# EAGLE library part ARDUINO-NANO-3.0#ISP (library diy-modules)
Arduino Nano 3.0 (and compatible devices) with ISP pads More details available here: https://www.arduino.cc/en/Main/ArduinoBoardNano Click here to find device on ebay.com
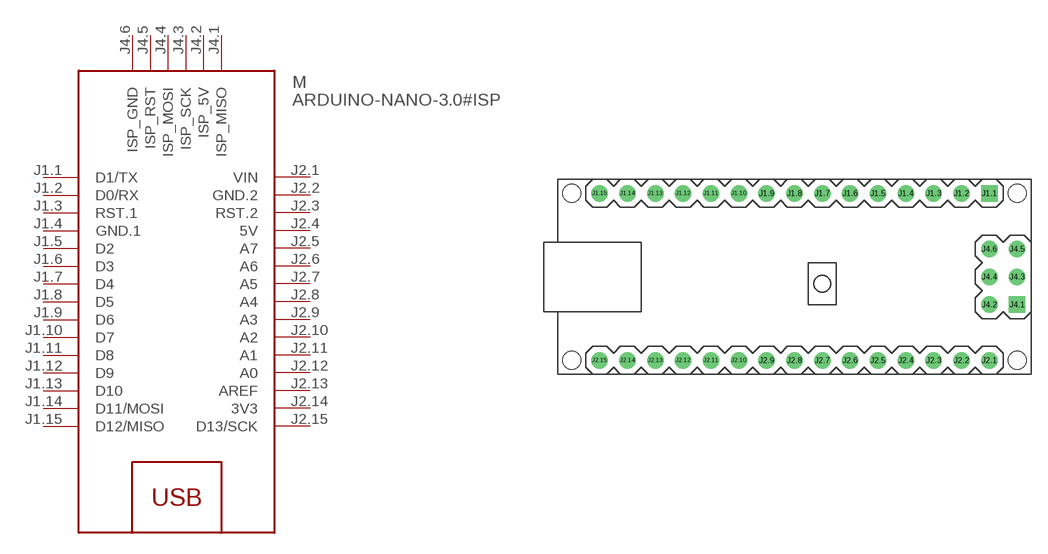
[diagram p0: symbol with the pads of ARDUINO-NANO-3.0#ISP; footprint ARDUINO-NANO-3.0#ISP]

Designator prefix M

## ARDUINO-NANO-3.0#ISP  [ARDUINO-NANO-3.0#ISP]
J1.1  D1/TX
J1.2  D0/RX
J1.3  RST.1
J1.4  GND.1  pwr
J1.5  D2
J1.6  D3
J1.7  D4
J1.8  D5
J1.9  D6
J1.10  D7
J1.11  D8
J1.12  D9
J1.13  D10
J1.14  D11/MOSI
J1.15  D12/MISO
J2.1  VIN  pwr
J2.2  GND.2  pwr
J2.3  RST.2
J2.4  5V  pwr
J2.5  A7
J2.6  A6
J2.7  A5
J2.8  A4
J2.9  A3
J2.10  A2
J2.11  A1
J2.12  A0
J2.13  AREF
J2.14  3V3  pwr
J2.15  D13/SCK
J4.1  ISP_MISO
J4.2  ISP_5V
J4.3  ISP_SCK
J4.4  ISP_MOSI
J4.5  ISP_RST
J4.6  ISP_GND

## Footprint ARDUINO-NANO-3.0#ISP (pad centres in mm)
Arduino Nano 3.0 Footprint with ISP pads
drill 1 square: J1.1 17.78,7.62; J4.1 20.32,-2.54
drill 1: J1.2 15.24,7.62; J1.3 12.7,7.62; J1.4 10.16,7.62; J1.5 7.62,7.62; J1.6 5.08,7.62; J1.7 2.54,7.62; J1.8 0,7.62; J1.9 -2.54,7.62; J1.10 -5.08,7.62; J1.11 -7.62,7.62; J1.12 -10.16,7.62; J1.13 -12.7,7.62; J1.14 -15.24,7.62; J1.15 -17.78,7.62; J2.1 17.78,-7.62; J2.2 15.24,-7.62; J2.3 12.7,-7.62; J2.4 10.16,-7.62; J2.5 7.62,-7.62; J2.6 5.08,-7.62; J2.7 2.54,-7.62; J2.8 0,-7.62; J2.9 -2.54,-7.62; J2.10 -5.08,-7.62; J2.11 -7.62,-7.62; J2.12 -10.16,-7.62; J2.13 -12.7,-7.62; J2.14 -15.24,-7.62; J2.15 -17.78,-7.62; J4.2 17.78,-2.54; J4.3 20.32,0; J4.4 17.78,0; J4.5 20.32,2.54; J4.6 17.78,2.54
hole 1.651 at -20.32,7.62
hole 1.651 at -20.32,-7.62
hole 1.651 at 20.32,-7.62
hole 1.651 at 20.32,7.62

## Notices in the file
Released under the Creative Commons Attribution 4.0 International License: http://creativecommons.org/licenses/by/4.0
